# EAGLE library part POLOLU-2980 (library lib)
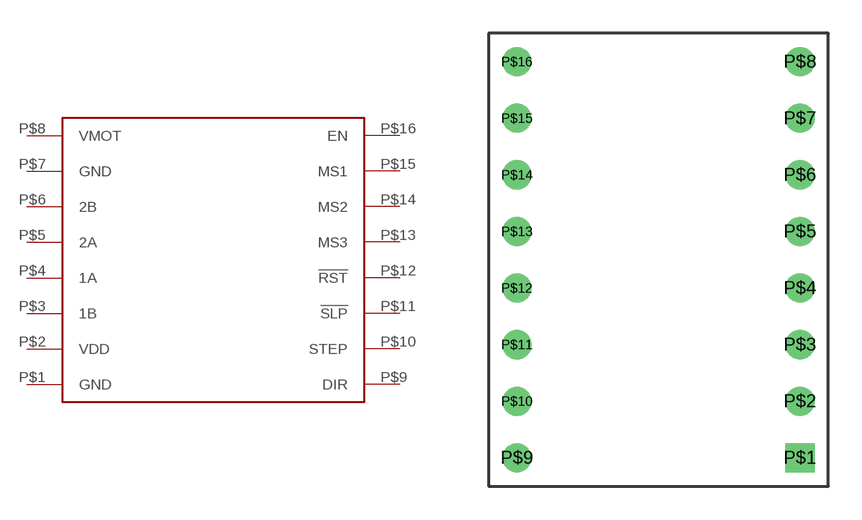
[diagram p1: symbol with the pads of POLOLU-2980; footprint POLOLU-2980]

Designator prefix -

## POLOLU-2980  [POLOLU-2980]
P$1  GND
P$2  VDD
P$3  1B
P$4  1A
P$5  2A
P$6  2B
P$7  GND
P$8  VMOT
P$9  DIR
P$10  STEP
P$11  !SLP
P$12  !RST
P$13  MS3
P$14  MS2
P$15  MS1
P$16  EN

## Footprint POLOLU-2980 (pad centres in mm)
drill 0.8 square: P$1 6.35,-8.89
drill 0.8: P$2 6.35,-6.35; P$3 6.35,-3.81; P$4 6.35,-1.27; P$5 6.35,1.27; P$6 6.35,3.81; P$7 6.35,6.35; P$8 6.35,8.89; P$9 -6.35,-8.89; P$10 -6.35,-6.35; P$11 -6.35,-3.81; P$12 -6.35,-1.27; P$13 -6.35,1.27; P$14 -6.35,3.81; P$15 -6.35,6.35; P$16 -6.35,8.89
